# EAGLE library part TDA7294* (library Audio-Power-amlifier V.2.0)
100V - 100W DMOS Audio Amplifier with Mute/Standby
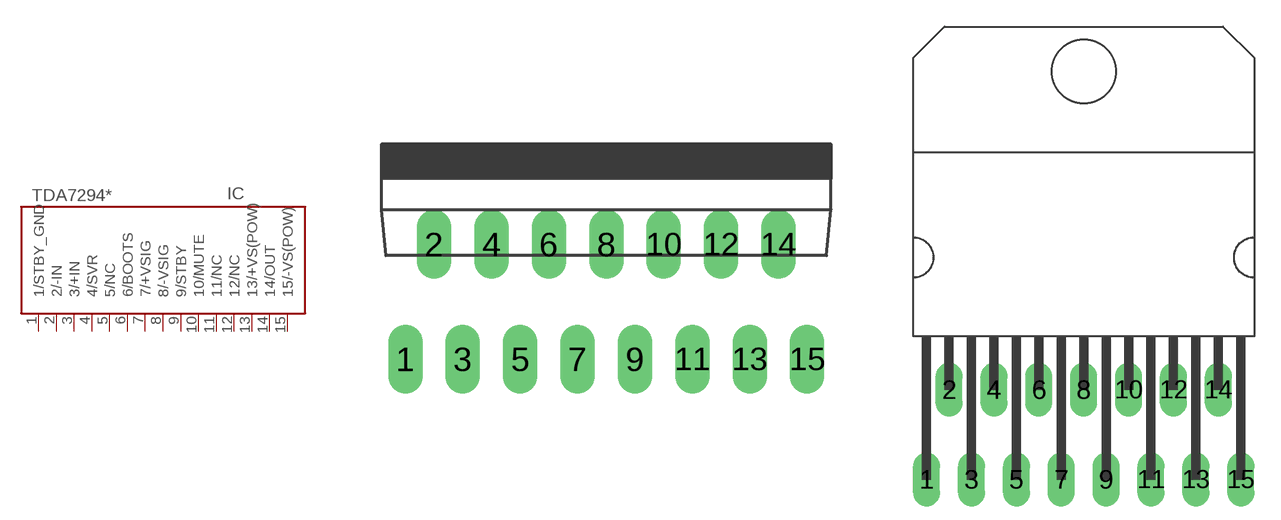
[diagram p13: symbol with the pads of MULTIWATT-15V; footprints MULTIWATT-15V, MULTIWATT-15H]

Designator prefix IC

## TDA7294VERTICAL  [MULTIWATT-15V]
1  1/STBY_GND  in
2  2/-IN  in
3  3/+IN  in
4  4/SVR
5  5/NC  nc
6  6/BOOTS
7  7/+VSIG  pwr
8  8/-VSIG  pwr
9  9/STBY  in
10  10/MUTE  in
11  11/NC  nc
12  12/NC  nc
13  13/+VS(POW)  pwr
14  14/OUT  out
15  15/-VS(POW)  pwr

## TDA7294HORIZONTAL  [MULTIWATT-15H]
Pads as for MULTIWATT-15V

## Footprint MULTIWATT-15V (pad centres in mm)
Multiwatt 15 vertical
drill 1.016 long: 1 -8.89,-5.08; 2 -7.62,0; 3 -6.35,-5.08; 4 -5.08,0; 5 -3.81,-5.08; 6 -2.54,0; 7 -1.27,-5.08; 8 0,0; 9 1.27,-5.08; 10 2.54,0; 11 3.81,-5.08; 12 5.08,0; 13 6.35,-5.08; 14 7.62,0; 15 8.89,-5.08

## Footprint MULTIWATT-15H (pad centres in mm)
Multiwatt 15 horizontal
drill 1.016 long: 1 -8.89,-5.08; 2 -7.62,0; 3 -6.35,-5.08; 4 -5.08,0; 5 -3.81,-5.08; 6 -2.54,0; 7 -1.27,-5.08; 8 0,0; 9 1.27,-5.08; 10 2.54,0; 11 3.81,-5.08; 12 5.08,0; 13 6.35,-5.08; 14 7.62,0; 15 8.89,-5.08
